PROGRAM MAIN
VAR
	fbModbusRTUMaster: ModbusRtuMaster_PcCOM;
	
	ModbusID: BYTE;
	ModbusQuantity: WORD;
	ModbusReadAddress: WORD;
	DataRead : ARRAY[1..15] OF REAL;
	bReadModbusData: BOOL;
	
	ModbusWriteAddress: WORD;
	DataWrite : DWORD;
	bWriteModbusData: BOOL;
END_VAR

//Reads data from a connected slave. Read Holding Registers
fbModbusRTUMaster.ReadRegs(
	UnitID:= ModbusID, 
	Quantity:= ModbusQuantity, 
	MBAddr:= ModbusReadAddress, 
	cbLength:= SIZEOF(DataRead), 
	pMemoryAddr:= ADR(DataRead), 
	Execute:= bReadModbusData, 
	Timeout:= T#3S, 
	BUSY=> , 
	Error=> , 
	ErrorId=> , 
	cbRead=> );

//Sends data to a connected slave
fbModbusRTUMaster.WriteRegs(
	UnitID:= ModbusID, 
	Quantity:= 1, 
	MBAddr:= ModbusWriteAddress, 
	cbLength:= SIZEOF(DataWrite), 
	pMemoryAddr:= ADR(DataWrite), 
	Execute:= bWriteModbusData, 
	Timeout:= , 
	BUSY=> , 
	Error=> , 
	ErrorId=> , 
	cbRead=> );

END_PROGRAM
